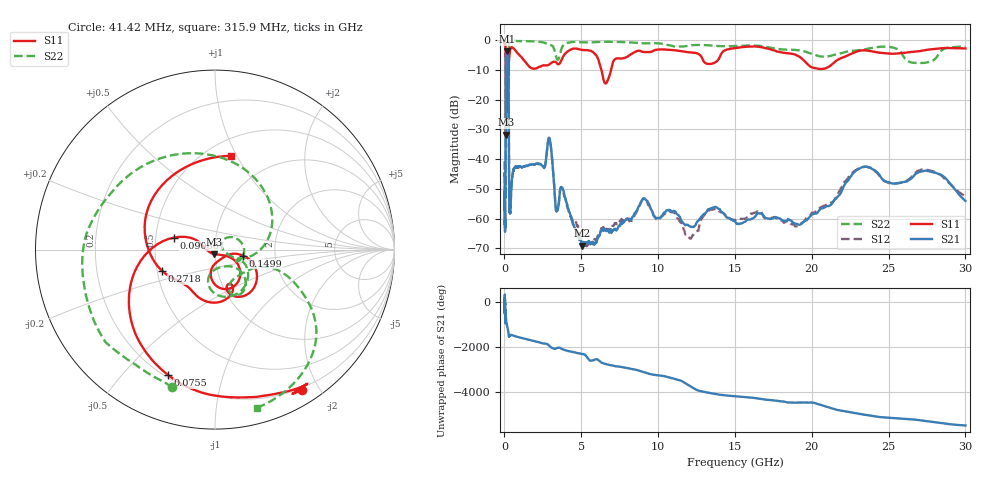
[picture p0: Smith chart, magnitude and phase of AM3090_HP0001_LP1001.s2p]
! Date/Time: Thu, Feb 28, 2019 1:54 PM
! Network Analyzer: Agilent Technologies E8364B Rev: A.07.50.67
! Sweep from 0.010 to 30.000 GHz, 1601 Points, Sweep Type: LOG
! Power Supply: 5.023 V, 0.002 A
# Hz S DB R 50
!freq MagS11 AngS11 MagS21 AngS21 MagS12 AngS12 MagS22 AngS22
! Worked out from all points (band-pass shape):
!   1601 points, 10 MHz to 30 GHz, reference 50 ohm
!   highest |S21| = -3.81 dB at 148.4 MHz (marker M1); lowest = -69.0 dB at 5.052 GHz (marker M2)
!   |S21| within 3 dB of the highest: 100.1 MHz to 248.8 MHz (148.7 MHz wide, 85.2 % of centre)
!   lowest |S11| = -31.8 dB at 98.93 MHz (marker M3), VSWR 1.05, Z = 49.5 - j2.5 ohm
!   |S11| at or under -10 dB: 89.61 MHz to 271.7 MHz (182.1 MHz wide, 101 % of centre); 6.309 GHz to 6.936 GHz (627.5 MHz wide, 9.47 % of centre)
!   |S22| runs from -27.7 to -0.1 dB; largest |S21 - S12| = 0.013
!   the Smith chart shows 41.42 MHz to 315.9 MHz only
!   S11 on the Smith chart (normalised r, x): 41.42 MHz: 0.17, -1.79; 75.5 MHz: 0.21, -0.67; 90.86 MHz: 0.62, +0.09; 149.9 MHz: 1.37, -0.09; 271.8 MHz: 0.53, -0.14; 315.9 MHz: 0.65, +0.95
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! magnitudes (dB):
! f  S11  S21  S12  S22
! 10 MHz  -0.2  -45.4  -40.7  -0.6
! 38.04 MHz  -0.5  -63.6  -60.3  -1.6
! 41.42 MHz  -0.7  -60.6  -61.7  -1.9
! 48.13 MHz  -0.9  -51.8  -47.6  -2.0
! 75.5 MHz  -2.5  -44.9  -43.2  -4.6
! 90.86 MHz  -12.5  -14.2  -14.2  -11.9
! 98.93 MHz  -31.8  -7.2  -7.2  -27.0
! 115 MHz  -12.9  -4.9  -4.8  -17.5
! 144.7 MHz  -20.6  -3.8  -3.8  -17.2
! 148.4 MHz  -17.0  -3.8  -3.8  -16.3
! 149.9 MHz  -15.9  -3.8  -3.8  -15.8
! 271.8 MHz  -10.0  -15.1  -15.1  -8.6
! 315.9 MHz  -5.5  -54.1  -56.4  -0.8
! 550.5 MHz  -2.7  -44.4  -44.4  -0.2
! 2.084 GHz  -9.5  -41.5  -41.5  -0.5
! 2.928 GHz  -8.1  -33.0  -33.0  -1.6
! 3.385 GHz  -7.6  -57.6  -57.3  -6.0
! 5.052 GHz  -3.3  -69.0  -69.1  -0.7
! 7.926 GHz  -5.8  -60.0  -60.4  -0.7
! 18.84 GHz  -4.7  -61.4  -62.0  -3.3
! 23.48 GHz  -3.5  -42.5  -42.5  -3.1
! 30 GHz  -2.8  -54.0  -52.5  -2.2
